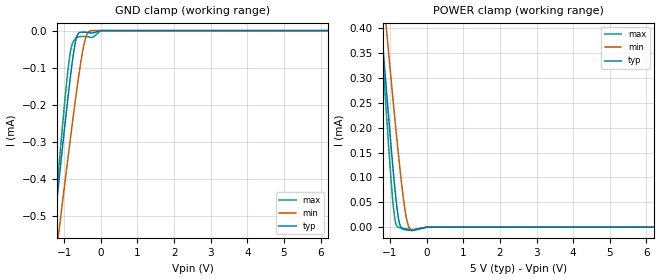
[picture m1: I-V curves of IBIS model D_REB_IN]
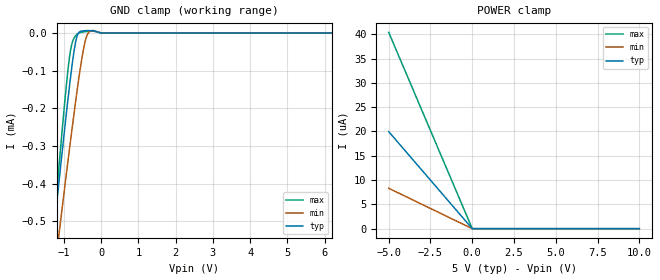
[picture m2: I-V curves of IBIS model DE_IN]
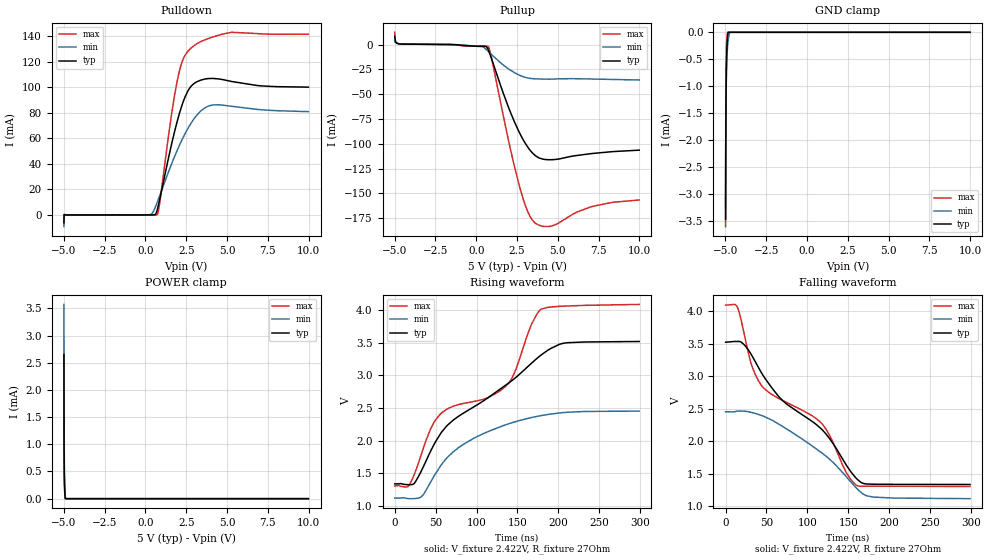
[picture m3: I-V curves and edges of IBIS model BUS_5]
| Texas Instruments Incorporated
| One, Two and Four Output, Integrated VCO, Low-Jitter Clock Generator
| Marketing part#   Voltage Range   Package-type   #pins/pkg drawing
| SN65HVD1781D   4.5V - 5.5V   D   8-pin SOIC
| SN65HVD1781DR   4.5V - 5.5V   D   8-pin SOIC
| SN65HVD1781DG4   4.5V - 5.5V   D   8-pin SOIC
| SN65HVD1781DRG4   4.5V - 5.5V   D   8-pin SOIC
[IBIS Ver]   4.0
[File name]   sn65hvd1781_5v.ibs
[File Rev]   1.1
[Date]   11/17/2010
[Source]   TISPICED simulations
   Texas Instruments Incorporated.
   Analog eLab Design Center, HPA
   12500 TI Blvd
   Dallas, TX -75243
   For Support e-mail: elab_scm_ibis@list.ti.com
[Notes]   Revision History:
   Rev 1.0: 05/14/2006
   - Initial version built by Industrial Interface Group
   Rev 1.1: 11/17/2010
   - Updated Disclaimer
   - updated IBIS ver to 4.0
   - Updated all models for Min and Max, revised typ
   - Ccomp for D_REB_in model has lower nom than min as a result of PVT corner
   - Ccomp for BUS_5 model has higher min than typ and lower max than typ due to PVT
   - Clamp current in RECEIVER_OUT model greater than 1A due to high operating voltage.
   - TISPice simulation of Clamp current does not match silicon
   - POWER and GND clamp for DE_IN, D_REB_IN non-monotonic due to low currents near 0V and TISpice
   - RECEIVER_OUT pullup/pulldown non-monotonic as a result of circuit design
[Disclaimer] This model is designed as an aid for customers of Texas Instruments.
 TI and its licensors and suppliers make no warranties, either expressed
 or implied, with respect to this  model, including the warranties of
 merchantability or fitness for a particular purpose.
 The model is provided solely on an "as is" basis. The entire risk as to
 its quality and performance is with the customer.
[Copyright] (C)Copyright 2010 Texas Instruments Incorporated.
   All rights reserved.
|   Component SN65VHD1781D
[Component]   SN65HVD1781D
[Manufacturer]  Texas Instruments Incorporated
[Package]   |SOIC (D) 8-pin
|   typ   min   max
R_pkg   0.103   0.061   0.136
L_pkg   1.993nH   1.693nH   2.314nH
C_pkg   0.373pF   0.352pF   0.398pF
[Pin]   signal_name   model_name   R_pin   L_pin   C_pin
1   R   RECEIVER_OUT   0.108   1.993n   0.363p
2   REB   D_REB_IN   0.103   1.929n   0.373p
3   DE   DE_IN   0.103   1.932n   0.373p
4   D   D_REB_IN   0.107   2.016n   0.352p
5   GND   GND   0.064   1.778n   0.394p
6   A   BUS_5   0.131   2.258n   0.391p
7   B   BUS_5   0.136   2.314n   0.391p
8   VCC   POWER   0.061   1.693n   0.398p
[Diff_pin]   inv_pin   vdiff   tdelay_typ   tdelay_min   tdelay_max
| The 'A' pin is Diff_pin and the 'B' pin is the inv_pin
6   7   0.200   0 0 0
| Models and submodels in the file (4): D_REB_IN (Input), DE_IN (Input), BUS_5 (I/O), RECEIVER_OUT (Output)
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|   Driver Input / Receiver Enable / Model
[Model]   D_REB_IN
Model_type   Input
|Signals   D,REB
Vinh = 2.0
Vinl = 0.8
| variable   typ   min   max
|   (slow PVT)   (nom PVT)   (fast PVT)
C_comp   .7253pF   .7251pF   .7755pF
| Ccomp comes from PVT
| Nom PVT: VCC=5.0V, Temp = 25C, models = nominal
| Slow PVT: VCC = 4.5V, Temp = 150C, models = weak
| Fast PVT: VCC = 5.5V, Temp = -40C, models = strong
|   typ   min   max
[Voltage Range]   5   4.5   5.5
[Temperature Range]   25   150   -40
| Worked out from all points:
|   GND clamp passes 1 mA (typ) near -1.76 V on its own axis
|   POWER clamp passes 1 mA (typ) near -1.86 V on its own axis
[GND Clamp]
| High Current due to TISpice simulations which do not match silicon
| High operating voltage drives high currents.
| Non-monotonic behavior is expected near 0V with small currents.
|   Voltage   I(typ)   I(min)   I(max)
-5V       -4.199mA   -3.819mA   -5.047mA
-1.288V   -540.4uA   -660.3uA   -531.7uA
-1.167V   -426.8uA   -561.5uA   -392.6uA
-1.085V   -349.6uA   -494.2uA   -299.1uA
-860mV    -148.4uA   -313.9uA   -75.45uA
-792.5mV  -94.06uA   -261.4uA   -39.98uA
-695mV    -31.25uA   -187.6uA   -21.54uA
-575mV    -5.063uA   -103.2uA   -16.16uA
-417.5mV  -4.458uA   -20.09uA   -16.21uA
-282.5mV  -5.924uA   -480.6nA   -17.87uA
0V        0A         0A         0A
10V       0A         0A         0A
[POWER Clamp]
| High Current due to TISpice simulations which do not match silicon
| High operating voltage drives high currents.
| Non-monotonic behavior is expected near 0V with small currents.
|   Voltage   I(typ)   I(min)   I(max)
-5V       4.107mA    3.706mA    4.957mA
-1.317V   479.8uA    576.1uA    478.9uA
-1.235V   402uA      508.6uA    383uA
-1.13V    304.2uA    423.5uA    263.2uA
-1.055V   235.9uA    363.4uA    180.6uA
-890mV    94.9uA     234.4uA    28.14uA
-837.5mV  56.21uA    194.8uA    6.165uA
-762.5mV  14.58uA    140.3uA    -444.4nA
-635mV    -4.429uA   57.46uA    -2.404uA
-515mV    -5.654uA   6.385uA    -3.959uA
-395mV    -6.533uA   -6.894uA   -5.377uA
10V       0A         0A         0A
|   Driver Enable / Model
[Model]   DE_IN
Model_type   Input
|Signals   DE
Vinh = 2.0
Vinl = 0.8
| variable   typ   min   max
C_comp   .7408pF   .7401pF   .792pF
[Voltage Range]   5   4.5   5.5
[Temperature Range]   25   150   -40
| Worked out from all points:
|   GND clamp passes 1 mA (typ) near -1.76 V on its own axis
[GND Clamp]
| High Current due to TISpice simulations which do not match silicon
| High operating voltage drives high currents.
| Non-monotonic behavior is expected near 0V with small currents.
|   Voltage   I(typ)   I(min)   I(max)
-5V       -4.2mA     -3.82mA    -5.047mA
-1.288V   -540.9uA   -660.9uA   -531.9uA
-1.272V   -526.6uA   -648.5uA   -514.3uA
-1.153V   -413uA     -549.9uA   -375.3uA
-1.085V   -349.9uA   -494.8uA   -298.7uA
-852.5mV  -141.5uA   -308.4uA   -65.26uA
-785mV    -87.18uA   -255.9uA   -27.95uA
-687.5mV  -23.95uA   -182.2uA   -7.117uA
-560mV    4.21uA     -92.85uA   1.088uA
-387.5mV  6.377uA    -7.762uA   4.151uA
-215mV    6.347uA    6.727uA    5.119uA
10V       0A         0A         0A
[POWER Clamp]
| Non-monotonic behavior is expected near 0V with small currents.
|   Voltage   I(typ)   I(min)   I(max)
-5V       19.96uA    8.308uA    40.38uA
0V        0A         0A         0A
5V        0A         0A         0A
10V       0A         0A         0A
|   BUS_5 Model
[Model]   BUS_5
Model_type   I/O
| Signals   A,B
Polarity   Non-Inverting
Enable   Active-High
Vinl = 0.9
Vinh = 1.7
Vmeas = 2.5
Vref = 2.5
Cref = 15pF
Rref = 27
| variable   typ   min   max
|   (nom PVT)   (fast PVT)   (slow PVT)
C_comp   17.63pF   8.599pF   19.73pF
| Ccomp comes from PVT corner simulations
| Nom PVT: VCC=5.0V, Temp = 25C, models = nominal
| Slow PVT: VCC = 4.5V, Temp = 150C, models = weak
| Fast PVT: VCC = 5.5V, Temp = -40C, models = strong
[Voltage Range]   5   4.5   5.5
[Temperature Range]   25   150   -40
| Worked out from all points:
|   slope of the pulldown table from 0 to 0.75 V, typ, clamps not added: 147 ohm
|   slope of the pullup table from 0 to 0.75 V, typ, clamps not added: 187 ohm
|   GND clamp passes 1 mA (typ) near -4.96 V on its own axis
|   POWER clamp passes 1 mA (typ) near -4.98 V on its own axis
|   falling waveform, V_fixture 2.422V, R_fixture 27Ohm: 20-80 % time 98.5ns typ, 77.4ns min, 111ns max; typ from 3.52 V to 1.34 V
|   rising waveform, V_fixture 2.422V, R_fixture 27Ohm: 20-80 % time 117ns typ, 78.7ns min, 125ns max; typ from 1.34 V to 3.52 V
[Pulldown]
|   Voltage   I(typ)   I(min)   I(max)
-4.992V   -6.232mA   -9.091mA   -2.161mA
-4.97V    187.6uA    -1.086mA   438.8uA
-4.933V   218.5uA    263.3uA    69.64uA
265mV     30.23uA    202.3uA    -14.83uA
730mV     4.151mA    10.05mA    427.7uA
872.5mV   11.83mA    14.95mA    8.727mA
1.645V    57.64mA    41.27mA    82.26mA
2.005V    75.88mA    52.26mA    108.3mA
2.38V     90.89mA    62.44mA    124mA
2.965V    102.9mA    75.11mA    132.6mA
4.188V    107mA      86.31mA    139.7mA
9.992V    100.2mA    81.02mA    141.8mA
[GND Clamp]
|   Voltage   I(typ)   I(min)   I(max)
-4.992V   -3.462mA   -3.267mA   -3.6mA
-4.985V   -2.385mA   -2.212mA   -2.183mA
-4.978V   -1.798mA   -1.752mA   -1.421mA
-4.97V    -1.4mA     -1.455mA   -967.7uA
-4.963V   -1.111mA   -1.234mA   -679.5uA
-4.947V   -727.9uA   -916uA     -375.1uA
-4.925V   -406.4uA   -607.2uA   -168.5uA
-4.895V   -189.4uA   -369.5uA   -54.41uA
-4.857V   -49.48uA   -212.1uA   0A
-4.835V   0A         -150.8uA   0A
-4.73V    0A         0A         0A
9.992V    0A         0A         0A
[Pullup]
|   Voltage   I(typ)   I(min)   I(max)
-4.992V   8.438mA    3.716mA    12.42mA
-4.947V   3.395mA    2.275mA    2.877mA
-4.745V   776.4uA    922uA      834.2uA
385mV     -1.688mA   -2.047mA   -1.552mA
752.5mV   -5.769mA   -7.084mA   -2.273mA
1.938V    -61.41mA   -24.01mA   -93.42mA
2.62V     -87.8mA    -30.61mA   -140.9mA
3.167V    -103.5mA   -33.65mA   -168.8mA
3.663V    -112.4mA   -34.57mA   -180.6mA
4.593V    -116.1mA   -34.87mA   -183.1mA
6.992V    -110.1mA   -34.67mA   -163.8mA
9.992V    -106.4mA   -35.67mA   -156.7mA
[POWER Clamp]
|   Voltage   I(typ)   I(min)   I(max)
-4.992V   2.652mA    3.574mA    1.929mA
-4.985V   1.172mA    1.661mA    948.6uA
-4.978V   726uA      1.034mA    583.2uA
-4.97V    495.9uA    712.3uA    385.7uA
-4.963V   353.6uA    516.3uA    265.1uA
-4.955V   256.6uA    384.3uA    186.2uA
-4.947V   186.1uA    289.2uA    131.8uA
-4.94V    132.6uA    217.6uA    92.61uA
-4.925V   55.95uA    116.6uA    40.36uA
-4.91V    3.667uA    48.81uA    7.088uA
-4.895V   0A         171.6nA    0A
9.992V    0A         0A         0A
[Ramp]
R_load = 27
|   typ   min   max
dV/dt_r   1.31057/6.93213e-07   0.800237/5.50779e-07   1.6707/7.04705e-07
dV/dt_f   1.31057/1.1184e-06   0.800237/9.31182e-07   1.6707/1.1806e-06
[Falling Waveform]
V_fixture = 2.422V
V_fixture_min = 1.763V
V_fixture_max = 2.696V
R_fixture = 27Ohm
C_fixture = 0F
|   Time   V(typ)   V(min)   V(max)
0s        3.521V     2.453V     4.09V
14.6ns    3.533V     2.464V     4.054V
31ns      3.341V     2.445V     3.201V
43.5ns    3.059V     2.399V     2.864V
69.6ns    2.626V     2.229V     2.628V
116.8ns   2.193V     1.829V     2.284V
148.1ns   1.625V     1.449V     1.509V
159ns     1.443V     1.295V     1.333V
180.7ns   1.341V     1.144V     1.311V
298.9ns   1.337V     1.119V     1.306V
[Rising Waveform]
V_fixture = 2.422V
V_fixture_min = 1.763V
V_fixture_max = 2.696V
R_fixture = 27Ohm
C_fixture = 0F
|   Time   V(typ)   V(min)   V(max)
0s        1.337V     1.119V     1.306V
17.9ns    1.323V     1.11V      1.324V
35.2ns    1.606V     1.174V     1.893V
56.5ns    2.117V     1.622V     2.416V
82.6ns    2.412V     1.932V     2.567V
139ns     2.882V     2.257V     2.88V
167.3ns   3.189V     2.355V     3.787V
178.9ns   3.313V     2.384V     4.017V
206.4ns   3.495V     2.431V     4.063V
298.9ns   3.521V     2.453V     4.09V
